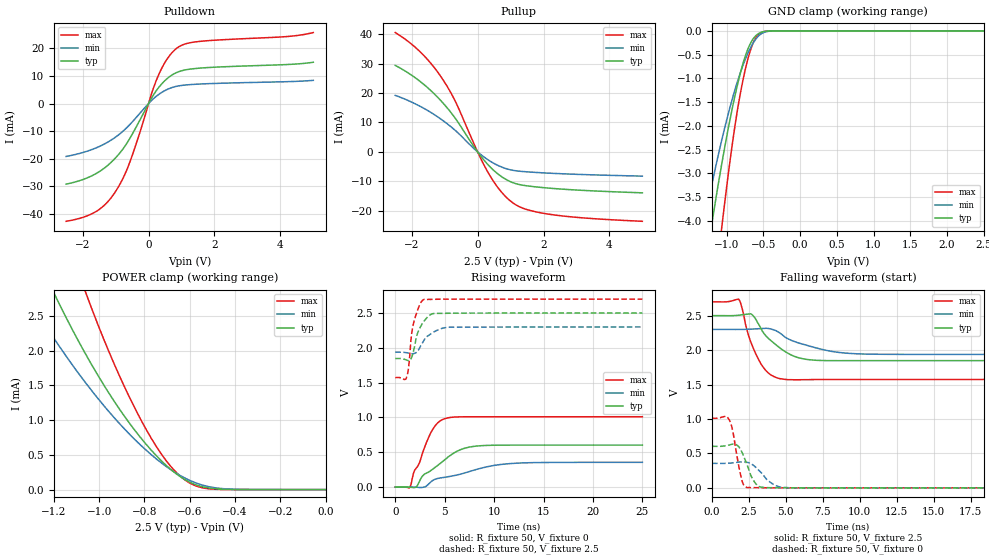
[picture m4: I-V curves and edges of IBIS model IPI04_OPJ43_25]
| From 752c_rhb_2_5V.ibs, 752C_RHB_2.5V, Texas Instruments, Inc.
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[Model]   IPI04_OPJ43_25
Model_type  I/O
Vinl = 0
Vinh = 2.5
Enable   Active-Low
Vref =   1.25
Rref =   50
Cref =   15p
Vmeas =   1.25
| variable   typ   min   max
C_comp   0.76pF   0.64pF   0.85pF
| C_pullup   1.93pF   0.63pF   2.89pF
| C_pulldown   1.74pF   0.87pF   2.69pF
| C_tri-state   0.76pF   0.64pF   0.85pF
[Temperature Range]   40   125   -40
| Ambient temperature   25   110   -40
[Voltage range]   2.5   2.3   2.7
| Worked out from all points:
|   slope of the pulldown table from 0 to 0.375 V, typ, clamps not added: 55.2 ohm
|   slope of the pullup table from 0 to 0.375 V, typ, clamps not added: 74 ohm
|   GND clamp passes 1 mA (typ) near -0.83 V on its own axis
|   POWER clamp passes 1 mA (typ) near -0.88 V on its own axis
|   rising waveform, R_fixture 50, V_fixture 0: 20-80 % time 3.28ns typ, 5.48ns min, 1.85ns max; typ from 0 V to 0.603 V
|   falling waveform, R_fixture 50, V_fixture 2.5: 20-80 % time 1.78ns typ, 2.71ns min, 1.14ns max; typ from 2.5 V to 1.85 V
|   rising waveform, R_fixture 50, V_fixture 2.5: 20-80 % time 953ps typ, 1.39ns min, 689ps max; typ from 1.85 V to 2.5 V
|   falling waveform, R_fixture 50, V_fixture 0: 20-80 % time 675ps typ, 979ps min, 503ps max; typ from 0.603 V to 0 V
[GND Clamp]
| IPI04_OPJ43_25
|   Voltage   I(typ)   I(min)   I(max)
-2.5V     -20.74mA   -15.76mA   -29.45mA
-1.32V    -5.285mA   -4.139mA   -7.815mA
-1.295V   -5.021mA   -3.943mA   -7.428mA
-1.195V   -4.005mA   -3.191mA   -5.931mA
-1.07V    -2.836mA   -2.326mA   -4.191mA
-1.05V    -2.661mA   -2.196mA   -3.929mA
-890mV    -1.395mA   -1.259mA   -2.04mA
-795mV    -788.5uA   -802.4uA   -1.175mA
-670mV    -249uA     -343.5uA   -383.2uA
-560mV    -53.09uA   -101.4uA   -68.45uA
-350mV    -679.5nA   -1.611uA   -400.1nA
2.5V      91.25pA    36.21nA    65.14pA
[POWER Clamp]
| IPI04_OPJ43_25
|   Voltage   I(typ)   I(min)   I(max)
-2.5V     16.04mA    11.67mA    23.13mA
-1.325V   3.727mA    2.827mA    5.527mA
-1.305V   3.578mA    2.719mA    5.302mA
-1.19V    2.767mA    2.133mA    4.079mA
-1.065V   1.983mA    1.561mA    2.889mA
-1.035V   1.81mA     1.434mA    2.626mA
-915mV    1.182mA    968.4uA    1.672mA
-810mV    720.6uA    619.9uA    971.2uA
-720mV    398uA      371.7uA    487.3uA
-630mV    161.7uA    181.2uA    161.2uA
-510mV    20.42uA    38.26uA    9.817uA
-31.11fV  91.25pA    390.6pA    73.39pA
[Pulldown]
| IPI04_OPJ43_25
|   Voltage   I(typ)   I(min)   I(max)
-2.5V     -29.18mA   -19.14mA   -42.63mA
-1.59V    -25.33mA   -16.04mA   -39.07mA
-1.275V   -22.74mA   -14.21mA   -36.02mA
-990mV    -19.52mA   -12.05mA   -31.63mA
-760mV    -16.15mA   -9.831mA   -26.67mA
-555mV    -12.34mA   -7.425mA   -20.77mA
100mV     2.15mA     1.22mA     3.901mA
285mV     5.465mA    3.101mA    9.823mA
560mV     9.001mA    5.082mA    16.06mA
855mV     11.25mA    6.26mA     20.03mA
1.49V     12.77mA    7.029mA    22.43mA
5V        14.96mA    8.404mA    25.71mA
[Pullup]
| IPI04_OPJ43_25
|   Voltage   I(typ)   I(min)   I(max)
-2.5V     29.41mA    19.22mA    40.58mA
-1.755V   24.05mA    15.55mA    34.15mA
-1.425V   20.9mA     13.45mA    30.19mA
-1.12V    17.47mA    11.19mA    25.69mA
-675mV    11.39mA    7.266mA    17.15mA
15mV      -232.4uA   -144.5uA   -367.9uA
300mV     -4.176mA   -2.587mA   -6.668mA
665mV     -7.939mA   -4.866mA   -12.86mA
1.035V    -10.32mA   -6.201mA   -17.06mA
1.455V    -11.49mA   -6.763mA   -19.48mA
2.19V     -12.36mA   -7.263mA   -21.25mA
5V        -13.94mA   -8.259mA   -23.63mA
[Ramp]
| IPI04_OPJ43_25
| variable   typ   min   max
dV/dt_r   0.37/3.29E-09   0.22/5.48E-09   0.61/1.87E-09
dV/dt_f   0.41/1.80E-09   0.23/2.79E-09   0.70/1.17E-09
R_load = 50
[Rising Waveform]
| IPI04_OPJ43_25
R_fixture =   50
C_fixture =   0
L_fixture =   0
V_fixture =   0
V_fixture_min = 0
V_fixture_max = 0
|   Time   V(typ)   V(min)   V(max)
0s        -6.212uV   -9.22uV    -2.898uV
1.47ns    -1.337mV   586uV      -4.923mV
2.115ns   -753.9uV   -1.792mV   271.4mV
2.785ns   163.1mV    -3.707mV   498.1mV
3.63ns    240.9mV    77.54mV    788.6mV
5.195ns   414.4mV    145.4mV    989.9mV
6.755ns   545.7mV    192mV      1.01V
8.685ns   594.8mV    271.8mV    1.01V
12.92ns   603.2mV    347.4mV    1.01V
24.99ns   603.3mV    355.9mV    1.01V
[Falling Waveform]
| IPI04_OPJ43_25
R_fixture =   50
C_fixture =   0
L_fixture =   0
V_fixture =   2.5
V_fixture_min = 2.3
V_fixture_max = 2.7
|   Time   V(typ)   V(min)   V(max)
0s        2.5V       2.3V       2.7V
1.81ns    2.506V     2.299V     2.739V
1.99ns    2.51V      2.3V       2.646V
2.63ns    2.526V     2.304V     2.116V
3.125ns   2.386V     2.309V     1.875V
3.78ns    2.178V     2.314V     1.674V
4.565ns   2.036V     2.252V     1.586V
6.235ns   1.87V      2.08V      1.57V
9.185ns   1.846V     1.953V     1.573V
24.99ns   1.847V     1.937V     1.573V
[Rising Waveform]
| IPI04_OPJ43_25
R_fixture =   50
C_fixture =   0
L_fixture =   0
V_fixture =   2.5
V_fixture_min = 2.3
V_fixture_max = 2.7
|   Time   V(typ)   V(min)   V(max)
0s        1.847V     1.937V     1.573V
1.145ns   1.826V     1.93V      1.575V
1.345ns   1.817V     1.924V     1.711V
1.605ns   1.846V     1.917V     2.135V
1.805ns   1.928V     1.915V     2.323V
2.24ns    2.202V     1.95V      2.532V
2.89ns    2.378V     2.103V     2.694V
3.745ns   2.489V     2.214V     2.697V
5.46ns    2.497V     2.296V     2.7V
24.99ns   2.5V       2.3V       2.7V
[Falling Waveform]
| IPI04_OPJ43_25
R_fixture =   50
C_fixture =   0
L_fixture =   0
V_fixture =   0
V_fixture_min = 0
V_fixture_max = 0
|   Time   V(typ)   V(min)   V(max)
0s        603.1mV    355.8mV    1.01V
1.18ns    622.9mV    358.6mV    982.9mV
1.4ns     634.7mV    362.6mV    832.8mV
2.035ns   515.6mV    377.6mV    101.1mV
2.39ns    327.7mV    370.4mV    3.238mV
2.715ns   144.1mV    340.1mV    3.488mV
3.15ns    23.75mV    259.9mV    2.875mV
3.955ns   2.218mV    79mV       791.4uV
4.785ns   1.851mV    7.083mV    187.5uV
24.99ns   1.484uV    1.024uV    523.5nV
